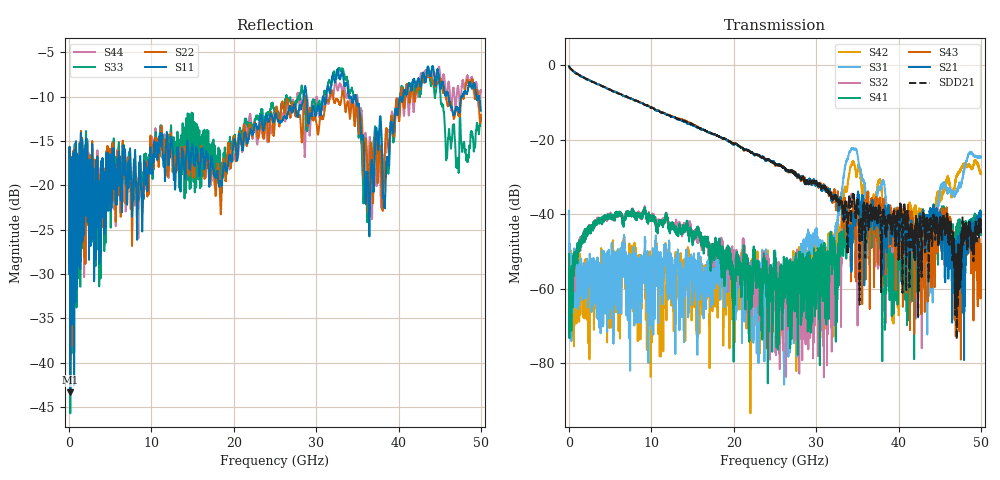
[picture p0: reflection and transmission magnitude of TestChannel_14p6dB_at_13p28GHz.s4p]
!Agilent Technologies,N5245A,MY49151038,A.09.90.19
!Agilent N5245A: A.09.90.19
!Date: Wednesday, February 07, 2018 06:27:35
!Correction: S11(Full 4 Port(1,2,3,4))
!S12(Full 4 Port(1,2,3,4))
!S13(Full 4 Port(1,2,3,4))
!S14(Full 4 Port(1,2,3,4))
!S21(Full 4 Port(1,2,3,4))
!S22(Full 4 Port(1,2,3,4))
!S23(Full 4 Port(1,2,3,4))
!S24(Full 4 Port(1,2,3,4))
!S31(Full 4 Port(1,2,3,4))
!S32(Full 4 Port(1,2,3,4))
!S33(Full 4 Port(1,2,3,4))
!S34(Full 4 Port(1,2,3,4))
!S41(Full 4 Port(1,2,3,4))
!S42(Full 4 Port(1,2,3,4))
!S43(Full 4 Port(1,2,3,4))
!S44(Full 4 Port(1,2,3,4))
!S4P File: Measurements: <S11,S12,S13,S14>,
!<S21,S22,S23,S24>,
!<S31,S32,S33,S34>,
!<S41,S42,S43,S44>:
# Hz S  MA  R 50
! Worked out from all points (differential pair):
!   5000 points, 10 MHz to 50 GHz, reference 50 ohm
!   strongest paths, dB at 10 MHz, 12.51 GHz, 25.01 GHz, 37.51 GHz, 50 GHz:
!     S21: -0.3, -13.9, -26.6, -40.3, -41.0
!     S43: -0.3, -13.8, -26.9, -51.0, -48.0
!     S41: -50.6, -42.4, -51.0, -42.2, -45.6
!     S32: -52.4, -43.1, -64.5, -52.1, -42.8
!     S31: -39.1, -53.7, -50.6, -33.4, -24.7
!     S42: -58.2, -56.5, -53.3, -31.6, -28.6
!   taken as a pair (ports 1,3 in; 2,4 out), SDD21 dB: -0.3, -13.8, -26.4, -41.0, -43.3
!   lowest |S11| = -43.4 dB at 150 MHz (marker M1), VSWR 1.01, Z = 49.3 + j0.141 ohm
!   |S11| at or under -10 dB: start of sweep to 28.5 GHz; 28.83 GHz to 30.81 GHz (1.975 GHz wide, 6.62 % of centre); 34.8 GHz to 40.2 GHz (5.4 GHz wide, 14.4 % of centre)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
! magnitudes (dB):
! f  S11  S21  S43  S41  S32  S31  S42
! 10 MHz  -30.0  -0.3  -0.3  -50.6  -52.4  -39.1  -58.2
! 150 MHz  -43.4  -0.8  -0.8  -64.7  -58.6  -60.2  -56.2
! 9.09 GHz  -18.8  -10.5  -10.5  -39.3  -39.4  -54.6  -55.2
! 27.75 GHz  -12.2  -29.8  -30.0  -66.5  -49.8  -67.2  -57.6
! 34.56 GHz  -10.3  -41.0  -37.3  -45.4  -38.3  -22.4  -26.0
! 43.8 GHz  -7.5  -39.2  -44.6  -45.1  -42.7  -56.3  -45.0
! 50 GHz  -11.6  -41.0  -48.0  -45.6  -42.8  -24.7  -28.6
